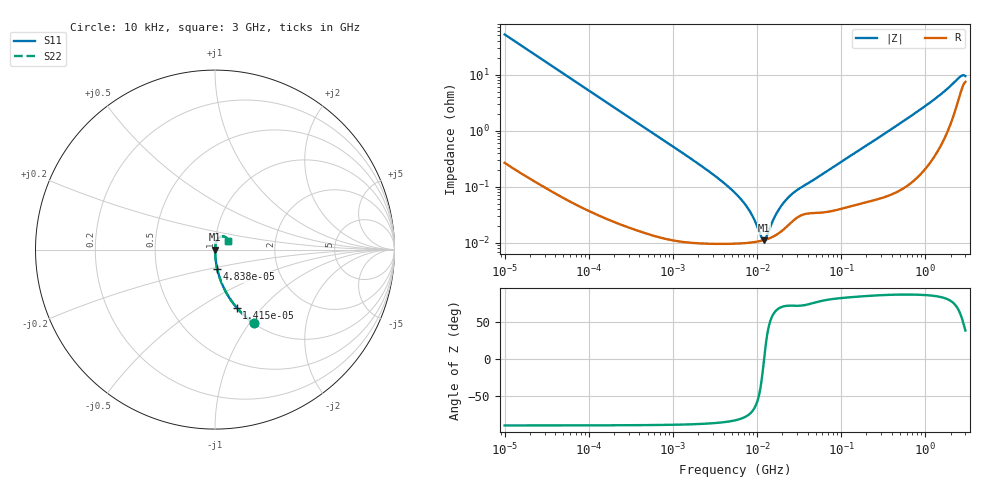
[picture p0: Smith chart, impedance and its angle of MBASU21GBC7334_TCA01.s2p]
! MBASU21GBC7334_TCA01  S-PARAMETER MODEL  ( Standard Model )
! Model Generated by TAIYO YUDEN Corporation (http://www.ty-top.com)
! Version 1.0
! TAIYO YUDEN Control No. 220601
! Copyright(c) 2014 TAIYO YUDEN CO.,LTD. All Rights Reserved.
! Product Description (link to TY-COMPAS)
! https://ds.yuden.co.jp/TYCOMPAS/or/detail?pn=MBASU21GBC7334KTCA01&u=M
! Products Name : Multilayer Ceramic Capacitors
! Characteristics :
!  Capacitance : 0.33 [uF] , Rated Voltage : 50 [V] , TCC : X7S
!  Case Size : 2.0 x 1.25 / 0.079 x 0.049 [mm/inch] , Thickness : 1.25 / 0.049 [mm/inch]
!  (Conditions: Temperature = 25 [degC] , DC Bias Voltage = 0 [V])
! External Node Assignments :
!  1  o---| |---o  2
! GND o---------o GND
! Frequency Range : 10kHz  -  3GHz  [ 401 STEP ]
# MHZ S RI R 50
! Freq[MHz].  S11 Real  S11 Imag  S21 Real  S21 Imag  S12 Real  S12 Imag  S22 Real  S22 Imag
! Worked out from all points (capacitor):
!   401 points, 10 kHz to 3 GHz, reference 50 ohm
!   read as one part in series: C = 305 nF near 10.65 kHz
!   lowest |Z| = 11.2 mohm at 12.05 MHz (marker M1)
!   series resonance near 12.15 MHz, so ESL is about 560 pH
!   S11 on the Smith chart (normalised r, x): 10 kHz: 1.01, -1.04; 14.15 kHz: 1.00, -0.74; 48.38 kHz: 1.00, -0.22; 3 GHz: 1.15, +0.12
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0.01  0.2148 -0.4081  0.7852 0.4081  0.7852 0.4081  0.2148 -0.4081
0.014146  0.121 -0.3236  0.879 0.3236  0.879 0.3236  0.121 -0.3236
0.023426  0.0484 -0.212  0.9516 0.212  0.9516 0.212  0.0484 -0.212
0.048377  0.0122 -0.1069  0.9878 0.1069  0.9878 0.1069  0.0122 -0.1069
0.082683  0.00443 -0.0631  0.9956 0.0631  0.9956 0.0631  0.00443 -0.0631
0.683653  0.000185 -0.00771  0.9998 0.00771  0.9998 0.00771  0.000185 -0.00771
2.737278  9.96e-05 -0.00184  0.9999 0.00184  0.9999 0.00184  9.96e-05 -0.00184
5.477226  9.72e-05 -0.000773  0.9999 0.000773  0.9999 0.000773  9.72e-05 -0.000773
6.829836  9.85e-05 -0.000533  0.9999 0.000533  0.9999 0.000533  9.85e-05 -0.000533
7.996027  0.0001 -0.000377  0.9999 0.000377  0.9999 0.000377  0.0001 -0.000377
9.361346  0.000103 -0.000231  0.9999 0.000231  0.9999 0.000231  0.000103 -0.000231
11.31085  0.000109 -6.29e-05  0.9999 6.29e-05  0.9999 6.29e-05  0.000109 -6.29e-05
12.04705  0.000112 -7.35e-06  0.9999 7.35e-06  0.9999 7.35e-06  0.000112 -7.35e-06
12.83117  0.000115 4.82e-05  0.9999 -4.82e-05  0.9999 -4.82e-05  0.000115 4.82e-05
17.04125  0.00014 0.000304  0.9999 -0.000304  0.9999 -0.000304  0.00014 0.000304
21.24962  0.000179 0.000513  0.9998 -0.000513  0.9998 -0.000513  0.000179 0.000513
28.22191  0.000264 0.000777  0.9997 -0.000777  0.9997 -0.000777  0.000264 0.000777
45.28751  0.00034 0.00123  0.9997 -0.00123  0.9997 -0.00123  0.00034 0.00123
374.4521  0.000804 0.01  0.9992 -0.01  0.9992 -0.01  0.000804 0.01
1240.86  0.00439 0.0346  0.9956 -0.0346  0.9956 -0.0346  0.00439 0.0346
2562.461  0.0457 0.0736  0.9543 -0.0736  0.9543 -0.0736  0.0457 0.0736
3000  0.0719 0.0501  0.9281 -0.0501  0.9281 -0.0501  0.0719 0.0501
